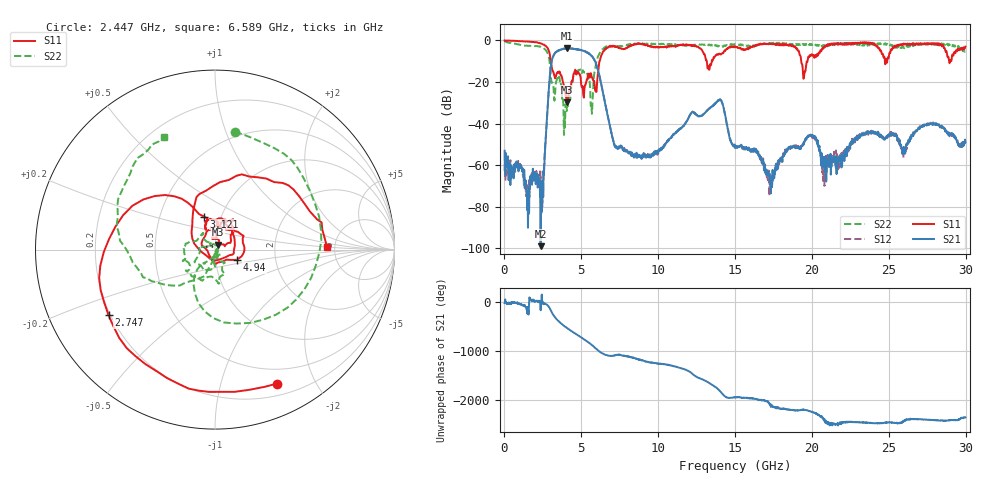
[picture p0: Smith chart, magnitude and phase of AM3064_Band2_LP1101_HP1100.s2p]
# Hz S DB R 50.0
!freq dBS11 angS11 dBS21 angS21 dBS12 angS12 dBS22 angS22
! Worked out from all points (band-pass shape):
!   1600 points, 10 MHz to 29.98 GHz, reference 50 ohm
!   highest |S21| = -3.76 dB at 4.059 GHz (marker M1); lowest = -98.9 dB at 2.353 GHz (marker M2)
!   |S21| within 3 dB of the highest: 3.226 GHz to 5.555 GHz (2.33 GHz wide, 53.1 % of centre); 5.56826 GHz to 5.57837 GHz (10.11 MHz wide, 0.181 % of centre)
!   lowest |S11| = -29.8 dB at 4.04 GHz (marker M3), VSWR 1.07, Z = 51.6 + j2.86 ohm
!   |S11| at or under -10 dB: 3.02 GHz to 6.186 GHz (3.166 GHz wide, 68.8 % of centre); 13.16 GHz to 13.48 GHz (326.7 MHz wide, 2.45 % of centre); 19.3 GHz to 19.71 GHz (406.2 MHz wide, 2.08 % of centre)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
!   |S22| runs from -45.5 to -0.3 dB; largest |S21 - S12| = 0.019
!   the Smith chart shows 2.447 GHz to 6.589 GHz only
!   S11 on the Smith chart (normalised r, x): 2.447 GHz: 0.33, -1.51; 2.747 GHz: 0.19, -0.27; 3.121 GHz: 0.83, +0.32; 4.94 GHz: 1.27, -0.15; 6.589 GHz: 4.32, +0.21
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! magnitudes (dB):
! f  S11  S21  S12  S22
! 10 MHz  0.0  -53.0  -62.8  -0.3
! 1.003 GHz  -0.4  -61.6  -59.3  -2.1
! 1.472 GHz  -0.6  -75.4  -74.1  -2.6
! 2.353 GHz  -1.4  -98.9  -72.2  -3.1
! 2.447 GHz  -1.7  -77.0  -70.0  -3.5
! 2.747 GHz  -3.1  -39.4  -39.4  -5.3
! 3.121 GHz  -14.2  -8.7  -8.5  -20.3
! 4.04 GHz  -29.8  -4.0  -3.8  -31.2
! 4.059 GHz  -29.1  -3.8  -3.8  -33.9
! 4.94 GHz  -17.3  -4.8  -4.7  -14.0
! 5.015 GHz  -21.9  -4.8  -4.7  -15.7
! 5.671 GHz  -17.5  -7.5  -7.5  -32.9
! 6.589 GHz  -4.1  -31.7  -31.6  -3.2
! 7.264 GHz  -3.1  -51.1  -50.9  -2.7
! 10 GHz  -3.4  -54.5  -53.4  -1.8
! 13.97 GHz  -6.4  -28.9  -28.7  -2.8
! 15 GHz  -2.9  -51.3  -51.8  -1.8
! 17.37 GHz  -1.7  -70.2  -65.2  -1.2
! 19.99 GHz  -6.7  -45.7  -45.7  -1.7
! 20.83 GHz  -3.4  -63.6  -61.3  -2.4
! 25 GHz  -8.0  -45.5  -45.3  -1.8
! 29.98 GHz  -3.0  -48.9  -49.6  -4.6
